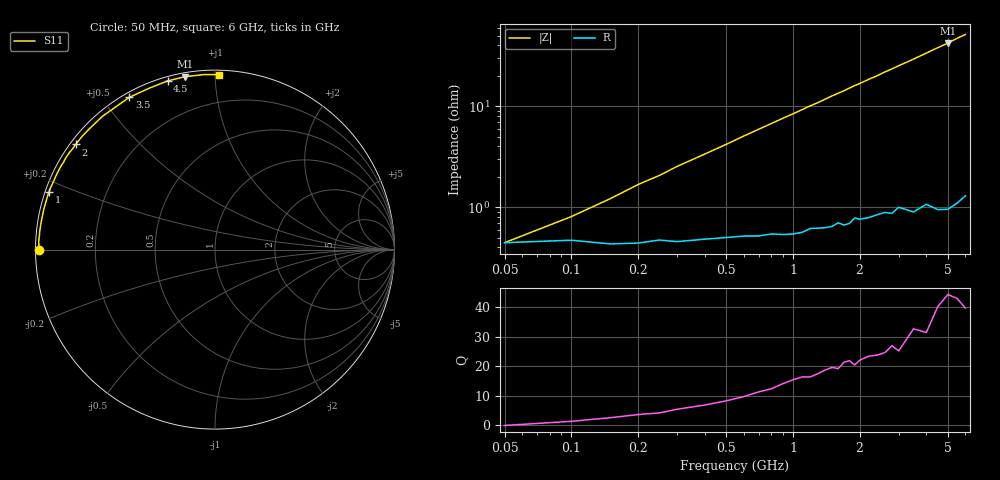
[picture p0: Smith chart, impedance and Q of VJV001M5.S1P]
! Infineon Technologies  Discrete & RF Semiconductors
! BB 914
! Si Tuning Diode in SOT23
! VR =
! S-Parameters:  July  1999
# GHz  S  MA  R  50
!  f  S11
! GHz  MAG  ANG
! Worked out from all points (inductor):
!   34 points, 50 MHz to 6 GHz, reference 50 ohm
!   read as one part to ground: L = 1.29 nH near 200 MHz
!   highest Q = 42.9 at 5 GHz (marker M1), where L = 1.34 nH
!   S11 on the Smith chart (normalised r, x): 50 MHz: 0.01, -0.00; 1 GHz: 0.01, +0.17; 2 GHz: 0.02, +0.33; 3.5 GHz: 0.02, +0.58; 4.5 GHz: 0.02, +0.76; 6 GHz: 0.03, +1.02
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0.05  0.9824 -180.0
0.1  0.9813 178.5
0.2  0.9826 176.3
0.25  0.9813 175.4
0.3  0.982 174.3
0.5  0.9803 170.5
0.6  0.9797 168.5
0.8  0.9789 164.7
1  0.9791 161.0
1.2  0.9766 157.2
1.3  0.9766 155.5
1.5  0.9761 151.7
1.6  0.9742 150.0
1.7  0.9757 148.3
1.8  0.975 146.4
1.9  0.972 144.6
2  0.973 143.0
2.2  0.9726 139.5
2.4  0.9714 136.4
2.6  0.9706 132.9
2.8  0.9719 129.9
3  0.9686 126.7
3.5  0.9736 119.4
4  0.9709 112.3
4.5  0.9762 105.7
5  0.9779 99.9
5.5  0.977 93.6
6  0.9751 88.6
